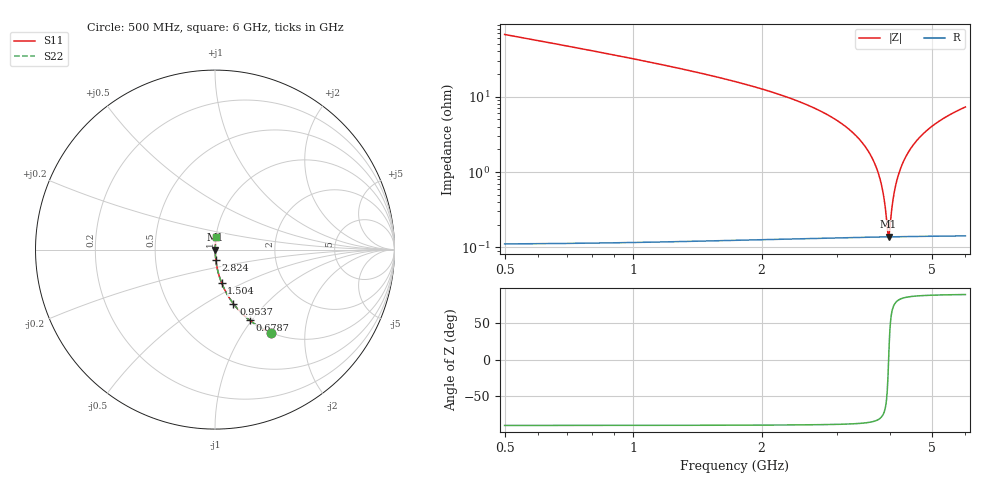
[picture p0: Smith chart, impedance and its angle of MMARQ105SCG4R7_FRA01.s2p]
! MMARQ105SCG4R7_FRA01  S-PARAMETER MODEL  ( General Type )
! Model Generated by TAIYO YUDEN Corporation (http://www.ty-top.com)
! Version 1.0
! TAIYO YUDEN Control No. 200326
! Copyright(c) 2020 TAIYO YUDEN CO.,LTD. All Rights Reserved.
! Product Description (link to TY-COMPAS)
! https://ds.yuden.co.jp/TYCOMPAS/or/detail?pn=MMARQ105SCG4R7BFRA01&u=M
! Products Name : Multilayer Ceramic Capacitors
! Characteristics :
!  Capacitance : 4.7 pF , Rated Voltage : 250V , TCC : CG / C0G
!  Case Size : 1.0 x 0.5 / 0.039 x 0.02 [mm/inch] , Thickness : 0.5 / 0.02 [mm/inch]
!  (Conditions: Temperature = 25 degC , DC Bias Current/Voltage = 0A / 0V)
! External Node Assignments :
!  1  o---| |---o  2
! GND o---------o GND
! Frequency Range : 500MHz  -  6GHz  [ 401 STEP ]
# MHz S RI R 50
! Freq[MHz].  S11 Real  S11 Imag  S21 Real  S21 Imag  S12 Real  S12 Imag  S22 Real  S22 Imag
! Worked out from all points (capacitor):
!   401 points, 500 MHz to 6 GHz, reference 50 ohm
!   read as one part in series: C = 4.67 pF near 527.5 MHz
!   lowest |Z| = 138 mohm at 3.965 GHz (marker M1)
!   series resonance near 3.966 GHz, so ESL is about 350 pH
!   S11 on the Smith chart (normalised r, x): 500 MHz: 1.00, -1.34; 678.8 MHz: 1.00, -0.98; 953.8 MHz: 1.00, -0.67; 1.504 GHz: 1.00, -0.39; 2.824 GHz: 1.00, -0.12; 6 GHz: 1.00, +0.15
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500  0.311 -0.4621  0.689 0.4621  0.689 0.4621  0.311 -0.4621
678.75  0.1927 -0.3933  0.8073 0.3933  0.8073 0.3933  0.1927 -0.3933
953.75  0.1027 -0.3019  0.8973 0.3019  0.8973 0.3019  0.1027 -0.3019
1421.25  0.0429 -0.1999  0.9571 0.1999  0.9571 0.1999  0.0429 -0.1999
1503.75  0.0374 -0.1866  0.9626 0.1866  0.9626 0.1866  0.0374 -0.1866
2342.5  0.0102 -0.0936  0.9898 0.0936  0.9898 0.0936  0.0102 -0.0936
2823.75  0.00484 -0.0591  0.9952 0.0591  0.9952 0.0591  0.00484 -0.0591
3250  0.00253 -0.0343  0.9975 0.0343  0.9975 0.0343  0.00253 -0.0343
3538.75  0.00175 -0.0196  0.9983 0.0196  0.9983 0.0196  0.00175 -0.0196
3731.25  0.00148 -0.0105  0.9985 0.0105  0.9985 0.0105  0.00148 -0.0105
3841.25  0.0014 -0.00548  0.9986 0.00548  0.9986 0.00548  0.0014 -0.00548
3882.5  0.00139 -0.00365  0.9986 0.00365  0.9986 0.00365  0.00139 -0.00365
3937.5  0.00138 -0.00124  0.9986 0.00124  0.9986 0.00124  0.00138 -0.00124
3965  0.00138 -4.3e-05  0.9986 4.3e-05  0.9986 4.3e-05  0.00138 -4.3e-05
3992.5  0.00138 0.00114  0.9986 -0.00114  0.9986 -0.00114  0.00138 0.00114
4075  0.0014 0.00465  0.9986 -0.00465  0.9986 -0.00465  0.0014 0.00465
4171.25  0.00146 0.00865  0.9985 -0.00865  0.9985 -0.00865  0.00146 0.00865
4308.75  0.00159 0.0142  0.9984 -0.0142  0.9984 -0.0142  0.00159 0.0142
4501.25  0.00187 0.0217  0.9981 -0.0217  0.9981 -0.0217  0.00187 0.0217
4762.5  0.00239 0.0315  0.9976 -0.0315  0.9976 -0.0315  0.00239 0.0315
5092.5  0.00328 0.0432  0.9967 -0.0432  0.9967 -0.0432  0.00328 0.0432
6000  0.00672 0.0726  0.9933 -0.0726  0.9933 -0.0726  0.00672 0.0726
